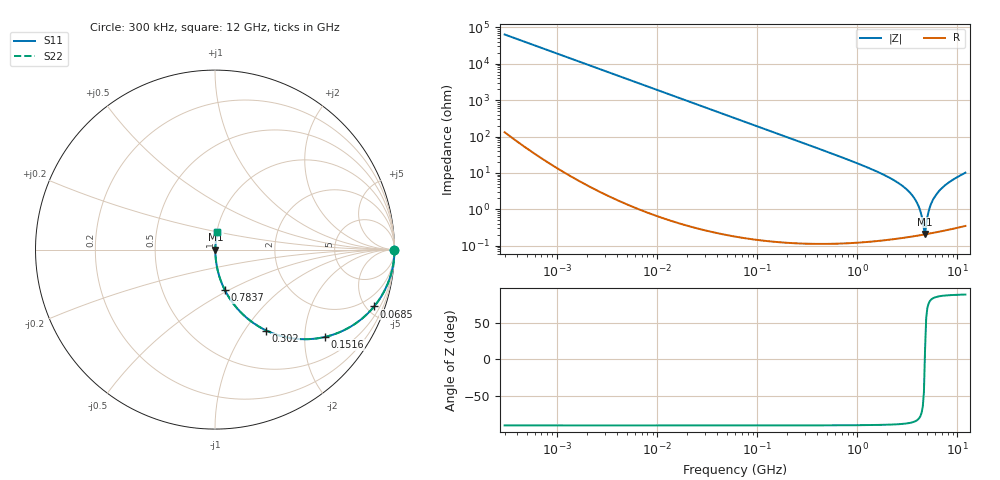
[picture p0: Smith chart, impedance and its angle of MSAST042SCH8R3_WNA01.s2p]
! MSAST042SCH8R3_WNA01  S-PARAMETER MODEL  ( General Type )
! Model Generated by TAIYO YUDEN Corporation (http://www.ty-top.com)
! Version 1.0
! TAIYO YUDEN Control No. 150820
! Copyright(c) 2015 TAIYO YUDEN CO.,LTD. All Rights Reserved.
! Product Description (link to TY-COMPAS)
! https://ds.yuden.co.jp/TYCOMPAS/or/detail?pn=MSAST042SCH8R3BWNA01&u=M
! Products Name : Multilayer Ceramic Capacitors
! Characteristics :
!  Capacitance : 8.3 pF , Rated Voltage : 25V , TCC : CH / C0H
!  Case Size : 0.4 x 0.2 / 0.016 x 0.008 [mm/inch] , Thickness : 0.2 / 0.008 [mm/inch]
!  (Conditions: Temperature = 25 degC , DC Bias Current/Voltage = 0A / 0V)
! External Node Assignments :
!  1  o---| |---o  2
! GND o---------o GND
! Frequency Range : 0.3MHz  -  12000MHz  [ 401 STEP ]
# MHz S RI R 50
! Freq[MHz].  S11 Real  S11 Imag  S21 Real  S21 Imag  S12 Real  S12 Imag  S22 Real  S22 Imag
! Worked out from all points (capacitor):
!   401 points, 300 kHz to 12 GHz, reference 50 ohm
!   read as one part in series: C = 8.3 pF near 316.3 kHz
!   lowest |Z| = 210 mohm at 4.748 GHz (marker M1)
!   series resonance near 4.723 GHz, so ESL is about 140 pH
!   S11 on the Smith chart (normalised r, x): 300 kHz: open; 68.5 MHz: 1.00, -5.60; 151.6 MHz: 1.00, -2.53; 302 MHz: 1.00, -1.26; 783.7 MHz: 1.00, -0.48; 12 GHz: 1.01, +0.20
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0.3  1 -0.00157  5.66e-06 0.00157  5.66e-06 0.00157  1 -0.00157
1.769972  0.9999 -0.00923  8.99e-05 0.00923  8.99e-05 0.00923  0.9999 -0.00923
10.44266  0.997 -0.0543  0.00298 0.0543  0.00298 0.0543  0.997 -0.0543
27.10171  0.9803 -0.1386  0.0197 0.1386  0.0197 0.1386  0.9803 -0.1386
60  0.9106 -0.285  0.0894 0.285  0.0894 0.285  0.9106 -0.285
68.49786  0.8866 -0.3168  0.1134 0.3168  0.1134 0.3168  0.8866 -0.3168
151.6462  0.6144 -0.4862  0.3856 0.4862  0.3856 0.4862  0.6144 -0.4862
301.9711  0.2859 -0.4509  0.7141 0.4509  0.7141 0.4509  0.2859 -0.4509
353.9943  0.2252 -0.4167  0.7748 0.4167  0.7748 0.4167  0.2252 -0.4167
783.7017  0.0545 -0.2247  0.9455 0.2247  0.9455 0.2247  0.0545 -0.2247
2088.533  0.00687 -0.0733  0.9931 0.0733  0.9931 0.0733  0.00687 -0.0733
2870.14  0.00341 -0.0421  0.9966 0.0421  0.9966 0.0421  0.00341 -0.0421
3547.679  0.00234 -0.0237  0.9977 0.0237  0.9977 0.0237  0.00234 -0.0237
4050.141  0.00205 -0.0127  0.998 0.0127  0.998 0.0127  0.00205 -0.0127
4270.516  0.00201 -0.00843  0.998 0.00843  0.998 0.00843  0.00201 -0.00843
4502.883  0.002 -0.00415  0.998 0.00415  0.998 0.00415  0.002 -0.00415
4747.894  0.00204 0.000502  0.998 -0.000502  0.998 -0.000502  0.00204 0.000502
4875.354  0.00207 0.00313  0.9979 -0.00313  0.9979 -0.00313  0.00207 0.00313
5420.343  0.00235 0.0134  0.9976 -0.0134  0.9976 -0.0134  0.00235 0.0134
6354.153  0.00318 0.0284  0.9968 -0.0284  0.9968 -0.0284  0.00318 0.0284
8281.503  0.0058 0.0551  0.9942 -0.0551  0.9942 -0.0551  0.0058 0.0551
12000  0.0135 0.0997  0.9865 -0.0997  0.9865 -0.0997  0.0135 0.0997
